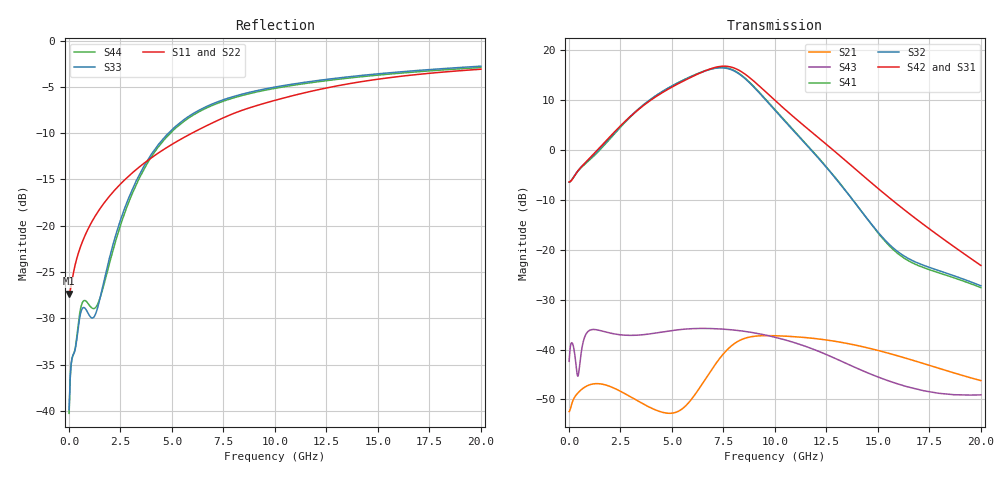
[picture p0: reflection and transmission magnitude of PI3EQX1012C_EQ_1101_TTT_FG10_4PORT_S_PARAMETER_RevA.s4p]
! NPort=4 DATA=2000 NOISE=0 GROUPDELAY=0 COMPLEX_DATAFORMAT=POLAR
! NumOfBlock=1 NumOfParam=0
! .MODEL Smodel S TSTONEFILE=PI3EQX1012C_EQ_1101_TTT_FG10_4PORT_S_PARAMETER_RevA.s4p TYPE=S
!  -- The above .MODEL line can be used for the S element in the netlist.
! The s parameter is extracted from the linear redriver, it is not bi-directional; only s(4,1)s(4,2) and s(3,1)s(3,2)
! should be the insertion loss
!Port definition:
!Port1 = input+
!Port2 = input-
!Port3 = output+
!Port4 = output-
# Hz S MA R  50
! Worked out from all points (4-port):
!   2000 points, 10 MHz to 20 GHz, reference 50 ohm
!   strongest paths, dB at 10 MHz, 5.01 GHz, 10.01 GHz, 15.01 GHz, 20 GHz:
!     S42: -6.4, 12.7, 9.9, -7.7, -23.1
!     S31: -6.4, 12.6, 9.9, -7.9, -23.6
!     S32: -6.4, 12.9, 7.9, -16.5, -27.2
!     S41: -6.4, 12.9, 8.1, -16.6, -27.6
!     S43: -42.4, -36.2, -37.5, -45.5, -49.1
!     S21: -52.4, -52.8, -37.2, -40.2, -46.2
!   lowest |S11| = -27.3 dB at 10 MHz (marker M1), VSWR 1.09, Z = 45.9 - j0.123 ohm
!   |S11| at or under -10 dB: start of sweep to 5.972 GHz
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1e7  0.04301 -178.2  0.002379 1.5  0.0008102 -0.5  0.0008039 -0.5
     0.002388 1.5  0.04109 -178.1  0.000927 -0.5  0.0009197 -0.5
     0.4787 0.4  0.4778 -179.5  0.01016 -4.0  0.007598 -25.7
     0.4773 -179.5  0.4796 0.4  0.007614 -25.8  0.009722 -4.0
4e9  0.2326 -124.3  0.002597 1.4  0.0003905 -56.3  0.0003886 -56.7
     0.002587 1.5  0.2361 -123.2  0.0004439 -57.0  0.0004417 -57.4
     3.198 -61.5  3.269 127.1  0.2432 -82.6  0.01343 34.9
     3.248 127.8  3.195 -59.8  0.01442 32.0  0.2354 -82.4
5.66e9  0.3029 -123.6  0.002815 52.1  0.0002818 -58.4  0.0002807 -59.3
        0.002712 49.9  0.3079 -122.9  0.0003196 -59.4  0.0003184 -60.2
        5.026 -129.9  5.146 58.4  0.3792 -98.7  0.01634 10.9
        5.161 58.7  5.047 -128.0  0.01604 8.2  0.3715 -98.4
6.95e9  0.3585 -124.2  0.006718 65.5  0.000242 -56.0  0.00024 -57.3
        0.006377 66.2  0.3638 -123.6  0.0002731 -57.2  0.000271 -58.5
        6.573 166.2  6.513 -6.1  0.4541 -108.8  0.01677 -9.4
        6.563 -6.1  6.611 168.3  0.01622 -10.1  0.4458 -108.7
8.02e9  0.4048 -125.7  0.01179 43.7  0.000226 -54.3  0.0002231 -55.8
        0.01142 45.2  0.4106 -125.2  0.0002534 -55.7  0.0002502 -57.1
        6.612 101.2  6.212 -71.5  0.4997 -115.4  0.01599 -24.2
        6.281 -71.9  6.654 103.5  0.01568 -24.3  0.4911 -115.3
9.23e9  0.4495 -127.9  0.01393 13.7  0.0002163 -53.8  0.0002125 -55.4
        0.01371 15.1  0.4563 -127.4  0.0002409 -55.0  0.0002367 -56.6
        4.385 33.6  3.769 -138.8  0.5396 -121.2  0.01462 -38.8
        3.823 -139.7  4.414 36.2  0.01439 -39.4  0.5309 -121.1
2e10  0.7002 -144.7  0.004945 -75.7  0.0001463 -72.3  0.0001411 -73.8
      0.004878 -74.9  0.7153 -144.4  0.0001622 -72.1  0.0001565 -73.8
      0.06634 101.5  0.04355 27.8  0.7272 -143.5  0.003594 -51.5
      0.04178 26.2  0.06964 106.2  0.003512 -48.8  0.7152 -143.3
